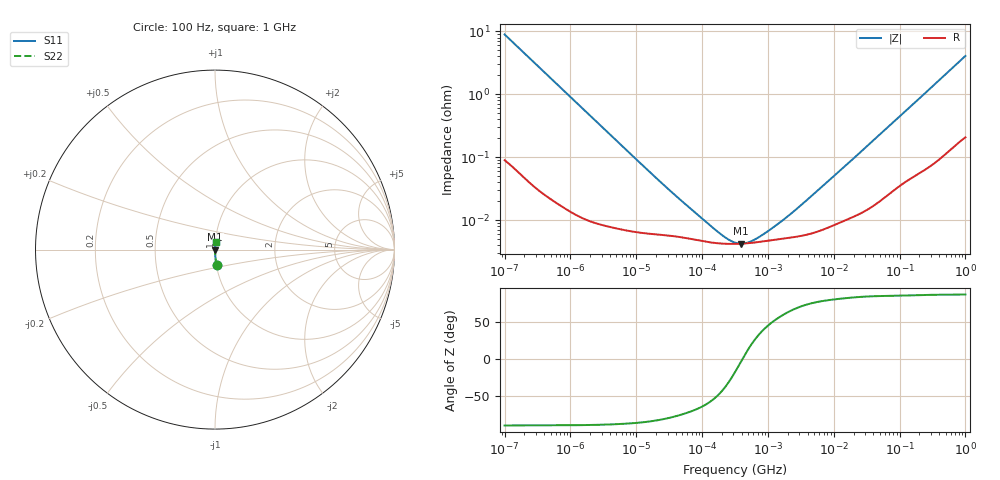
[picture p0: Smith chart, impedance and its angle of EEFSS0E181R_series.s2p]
!  *** S-Parameter ***
!  Copyright (C) Panasonic Industry Corporation
!  Conductive Polymer Aluminum Electrolytic Capacitor (SP-Cap)
!  Parts No. EEFSS0E181R
!  Connection Mode : Series
!  1  o---||---o  2
!  GND o--------o GND
!  Conditions : Temperature = 20 degC , DC Bias = 0 V
! Frequency Range : 100Hz  -  1GHz  [ 401 Steps ]
# Hz S RI R 50
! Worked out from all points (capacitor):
!   401 points, 100 Hz to 1 GHz, reference 50 ohm
!   read as one part in series: C = 178 uF near 108.4 Hz
!   lowest |Z| = 4.21 mohm at 386.8 kHz (marker M1)
!   series resonance near 409.6 kHz, so ESL is about 850 pH
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100  0.00881 -0.0886  0.9912 0.0886  0.9912 0.0886  0.00881 -0.0886
108.3927  0.00759 -0.0819  0.9924 0.0819  0.9924 0.0819  0.00759 -0.0819
175.7924  0.00313 -0.0509  0.9969 0.0509  0.9969 0.0509  0.00313 -0.0509
296.8247  0.00124 -0.0303  0.9988 0.0303  0.9988 0.0303  0.00124 -0.0303
588.8437  0.000427 -0.0153  0.9996 0.0153  0.9996 0.0153  0.000427 -0.0153
1487.647  0.000145 -0.00611  0.9999 0.00611  0.9999 0.00611  0.000145 -0.00611
22130.95  5.86e-05 -0.00042  0.9999 0.00042  0.9999 0.00042  5.86e-05 -0.00042
45708.82  5.37e-05 -0.000207  0.9999 0.000207  0.9999 0.000207  5.37e-05 -0.000207
102329.3  4.61e-05 -9.26e-05  1 9.26e-05  1 9.26e-05  4.61e-05 -9.26e-05
115478.2  4.51e-05 -8.1e-05  1 8.1e-05  1 8.1e-05  4.51e-05 -8.1e-05
316227.8  4.17e-05 -1.32e-05  1 1.32e-05  1 1.32e-05  4.17e-05 -1.32e-05
386812.1  4.2e-05 -2.85e-06  1 2.85e-06  1 2.85e-06  4.2e-05 -2.85e-06
1522299  4.98e-05 7.68e-05  1 -7.68e-05  1 -7.68e-05  4.98e-05 7.68e-05
1650061  5.03e-05 8.37e-05  0.9999 -8.37e-05  0.9999 -8.37e-05  5.03e-05 8.37e-05
1788546  5.09e-05 9.1e-05  0.9999 -9.1e-05  0.9999 -9.1e-05  5.09e-05 9.1e-05
2101358  5.21e-05 0.000107  0.9999 -0.000107  0.9999 -0.000107  5.21e-05 0.000107
4704354  6.15e-05 0.000239  0.9999 -0.000239  0.9999 -0.000239  6.15e-05 0.000239
1.778279e7  0.000107 0.000846  0.9999 -0.000846  0.9999 -0.000846  0.000107 0.000846
6.99842e7  0.00027 0.00315  0.9997 -0.00315  0.9997 -0.00315  0.00027 0.00315
3.368992e8  0.000998 0.0142  0.999 -0.0142  0.999 -0.0142  0.000998 0.0142
9.225714e8  0.00334 0.0374  0.9967 -0.0374  0.9967 -0.0374  0.00334 0.0374
1e9  0.0037 0.0404  0.9963 -0.0404  0.9963 -0.0404  0.0037 0.0404
